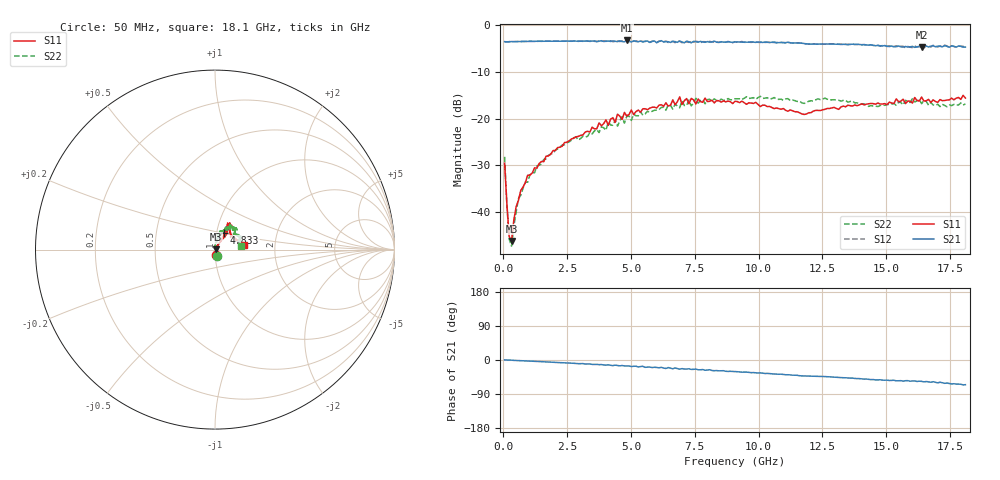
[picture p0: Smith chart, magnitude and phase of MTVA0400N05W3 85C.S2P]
! Network Analyzer HP8720D.06.14 Serial No. US36140669
!  8 Jul 2005  06:42:05
! Frequency  S11  S21  S12  S22
# HZ  S  DB R 50
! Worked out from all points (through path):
!   201 points, 50 MHz to 18.1 GHz, reference 50 ohm
!   highest |S21| = -3.30 dB at 4.833 GHz (marker M1); lowest = -4.8 dB at 16.39 GHz (marker M2)
!   group delay of S21, straight-line fit = 10 ps
!   lowest |S11| = -46.1 dB at 320.8 MHz (marker M3), VSWR 1.01, Z = 50.4 + j0.221 ohm
!   |S11| at or under -10 dB: start of sweep to end of sweep
!   |S22| runs from -47.3 to -15.2 dB; largest |S21 - S12| = 0.029
!   S11 on the Smith chart (normalised r, x): 50 MHz: 1.01, -0.07; 4.833 GHz: 1.08, +0.21; 18.1 GHz: 1.39, +0.07
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5e7  -29.54 -78.4  -3.55 0.3  -3.56 0.4  -28.16 -73.8
1.4025e8  -38.35 -68.9  -3.62 -0.0  -3.60 -0.1  -38.60 -108.6
2.305e8  -45.21 -35.7  -3.56 -0.3  -3.55 -0.3  -45.77 -142.8
3.2075e8  -46.14 26.4  -3.53 -0.4  -3.55 -0.4  -47.26 139.5
4.11e8  -41.70 45.1  -3.56 -1.0  -3.54 -0.9  -43.04 115.4
5.915e8  -37.46 57.7  -3.52 -1.2  -3.54 -1.3  -37.10 96.9
1.04275e9  -32.09 62.8  -3.48 -2.9  -3.49 -2.9  -32.00 81.5
1.94525e9  -26.84 57.0  -3.47 -5.9  -3.46 -5.9  -27.47 77.7
3.1185e9  -23.49 56.7  -3.45 -9.5  -3.48 -9.9  -23.76 78.6
4.021e9  -20.27 57.4  -3.46 -13.5  -3.47 -12.6  -22.50 73.2
4.11125e9  -21.44 57.3  -3.42 -12.6  -3.49 -13.7  -20.71 72.8
4.47225e9  -19.05 53.5  -3.55 -14.6  -3.39 -14.0  -21.61 76.7
4.83325e9  -19.43 62.2  -3.30 -15.8  -3.47 -16.3  -19.55 65.6
6.09675e9  -17.14 58.0  -3.52 -20.6  -3.42 -20.4  -18.08 64.1
6.7285e9  -17.06 63.5  -3.54 -21.0  -3.77 -21.6  -16.91 57.0
6.909e9  -15.35 61.2  -3.41 -24.2  -3.47 -22.6  -17.68 56.8
6.99925e9  -16.98 60.5  -3.62 -22.7  -3.78 -24.3  -16.22 57.8
9.075e9  -16.29 57.9  -3.62 -30.6  -3.59 -30.7  -15.77 48.3
1.21435e10  -18.39 38.0  -4.08 -42.4  -4.02 -42.6  -16.25 49.7
1.512175e10  -16.48 5.2  -4.59 -54.2  -4.42 -54.0  -16.95 36.7
1.638525e10  -15.39 4.7  -4.78 -56.4  -4.52 -56.1  -16.81 23.0
1.81e10  -15.60 8.9  -4.72 -65.2  -4.82 -65.2  -16.84 7.9
